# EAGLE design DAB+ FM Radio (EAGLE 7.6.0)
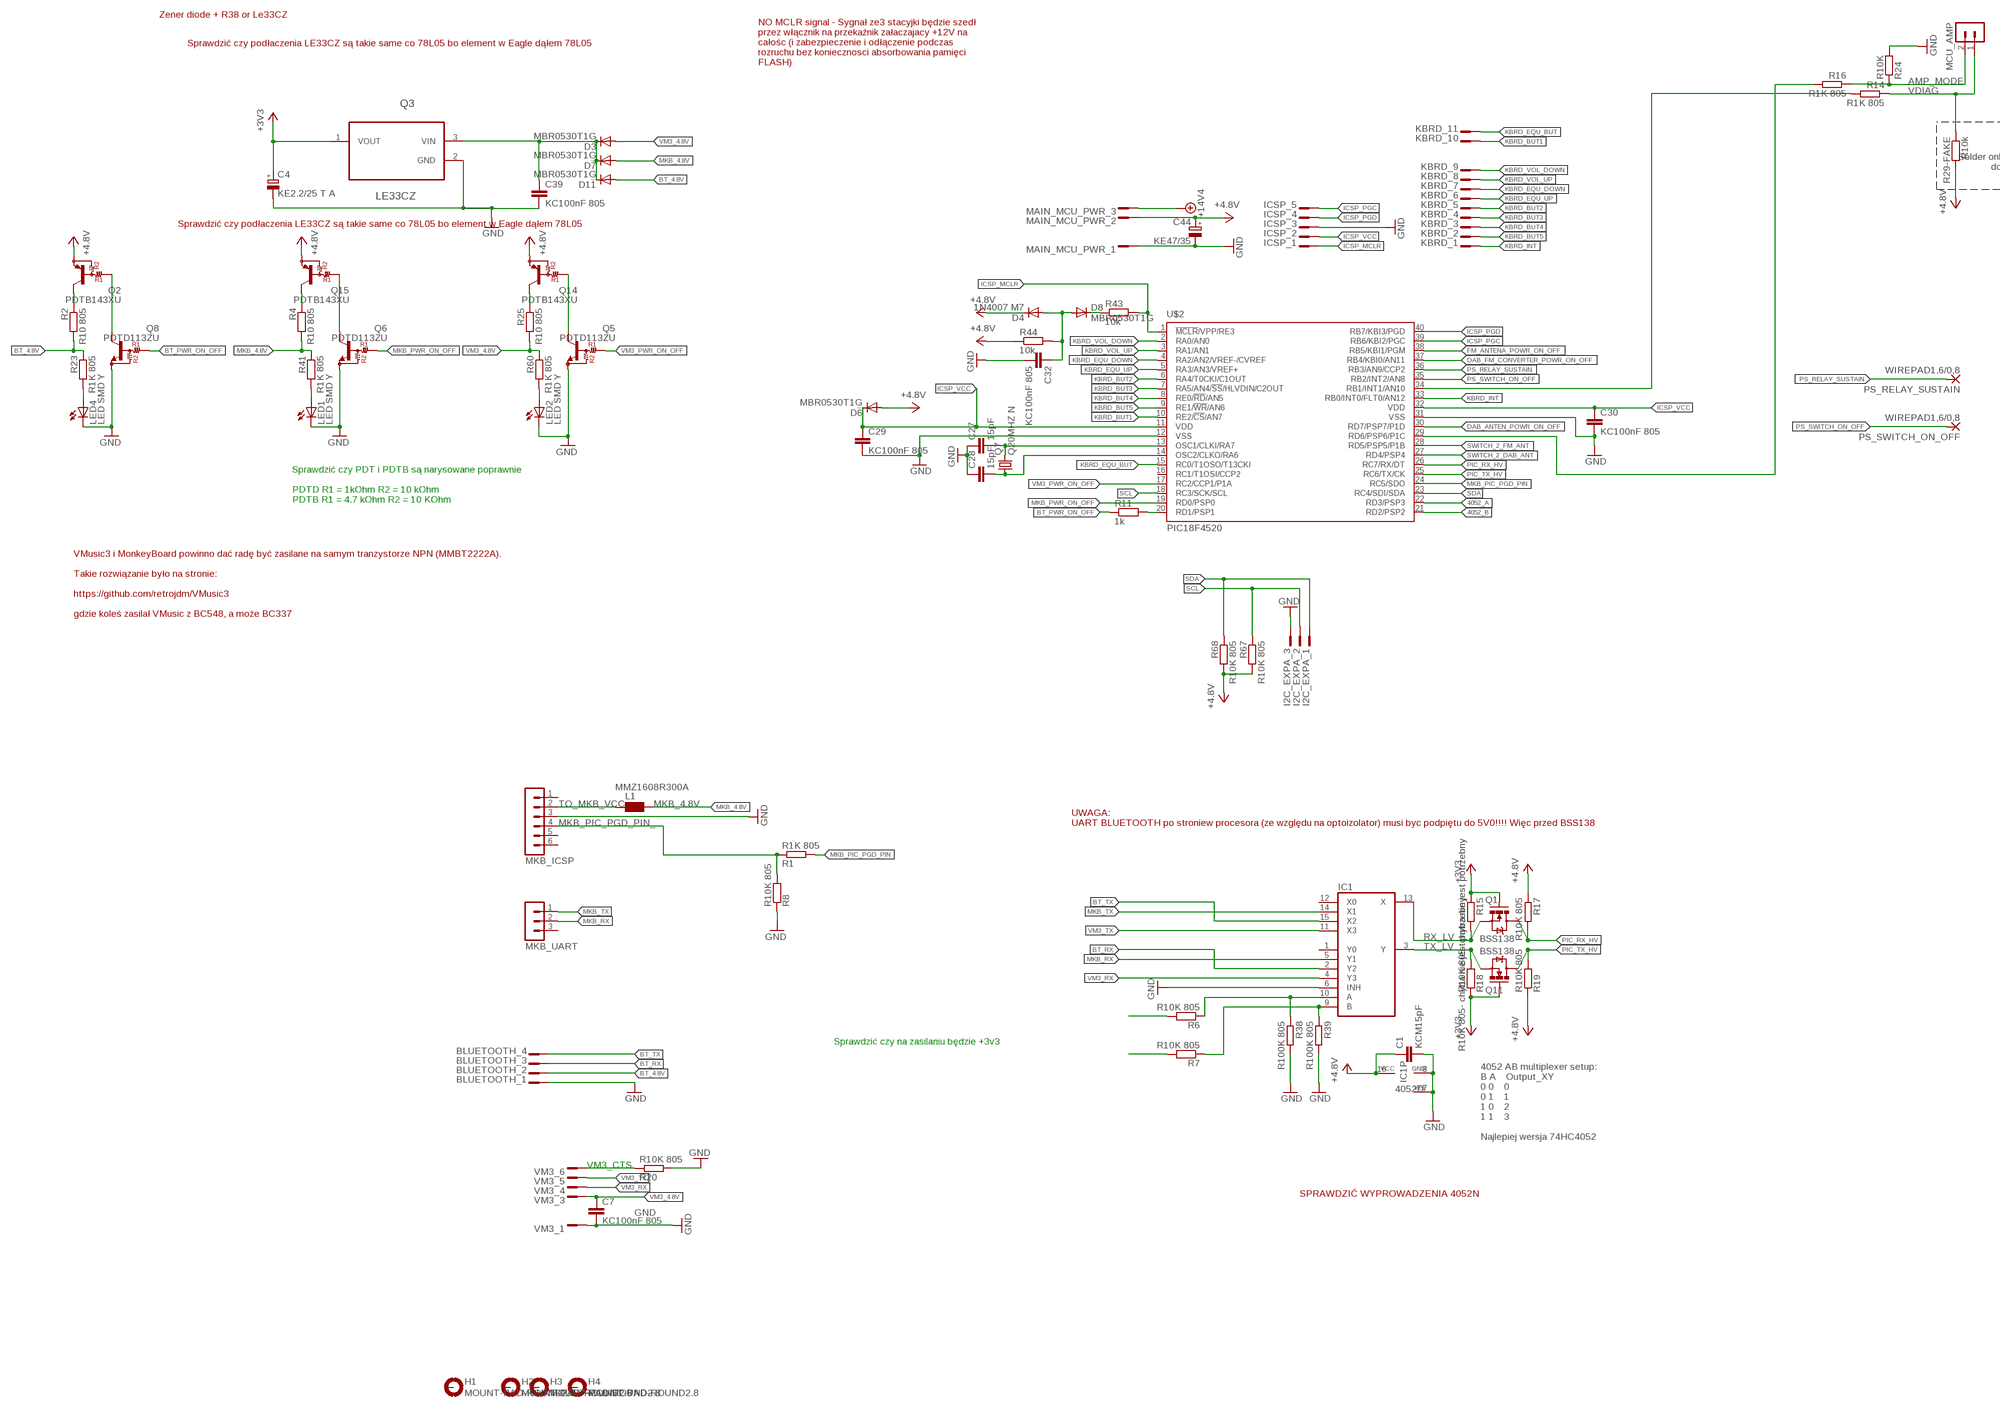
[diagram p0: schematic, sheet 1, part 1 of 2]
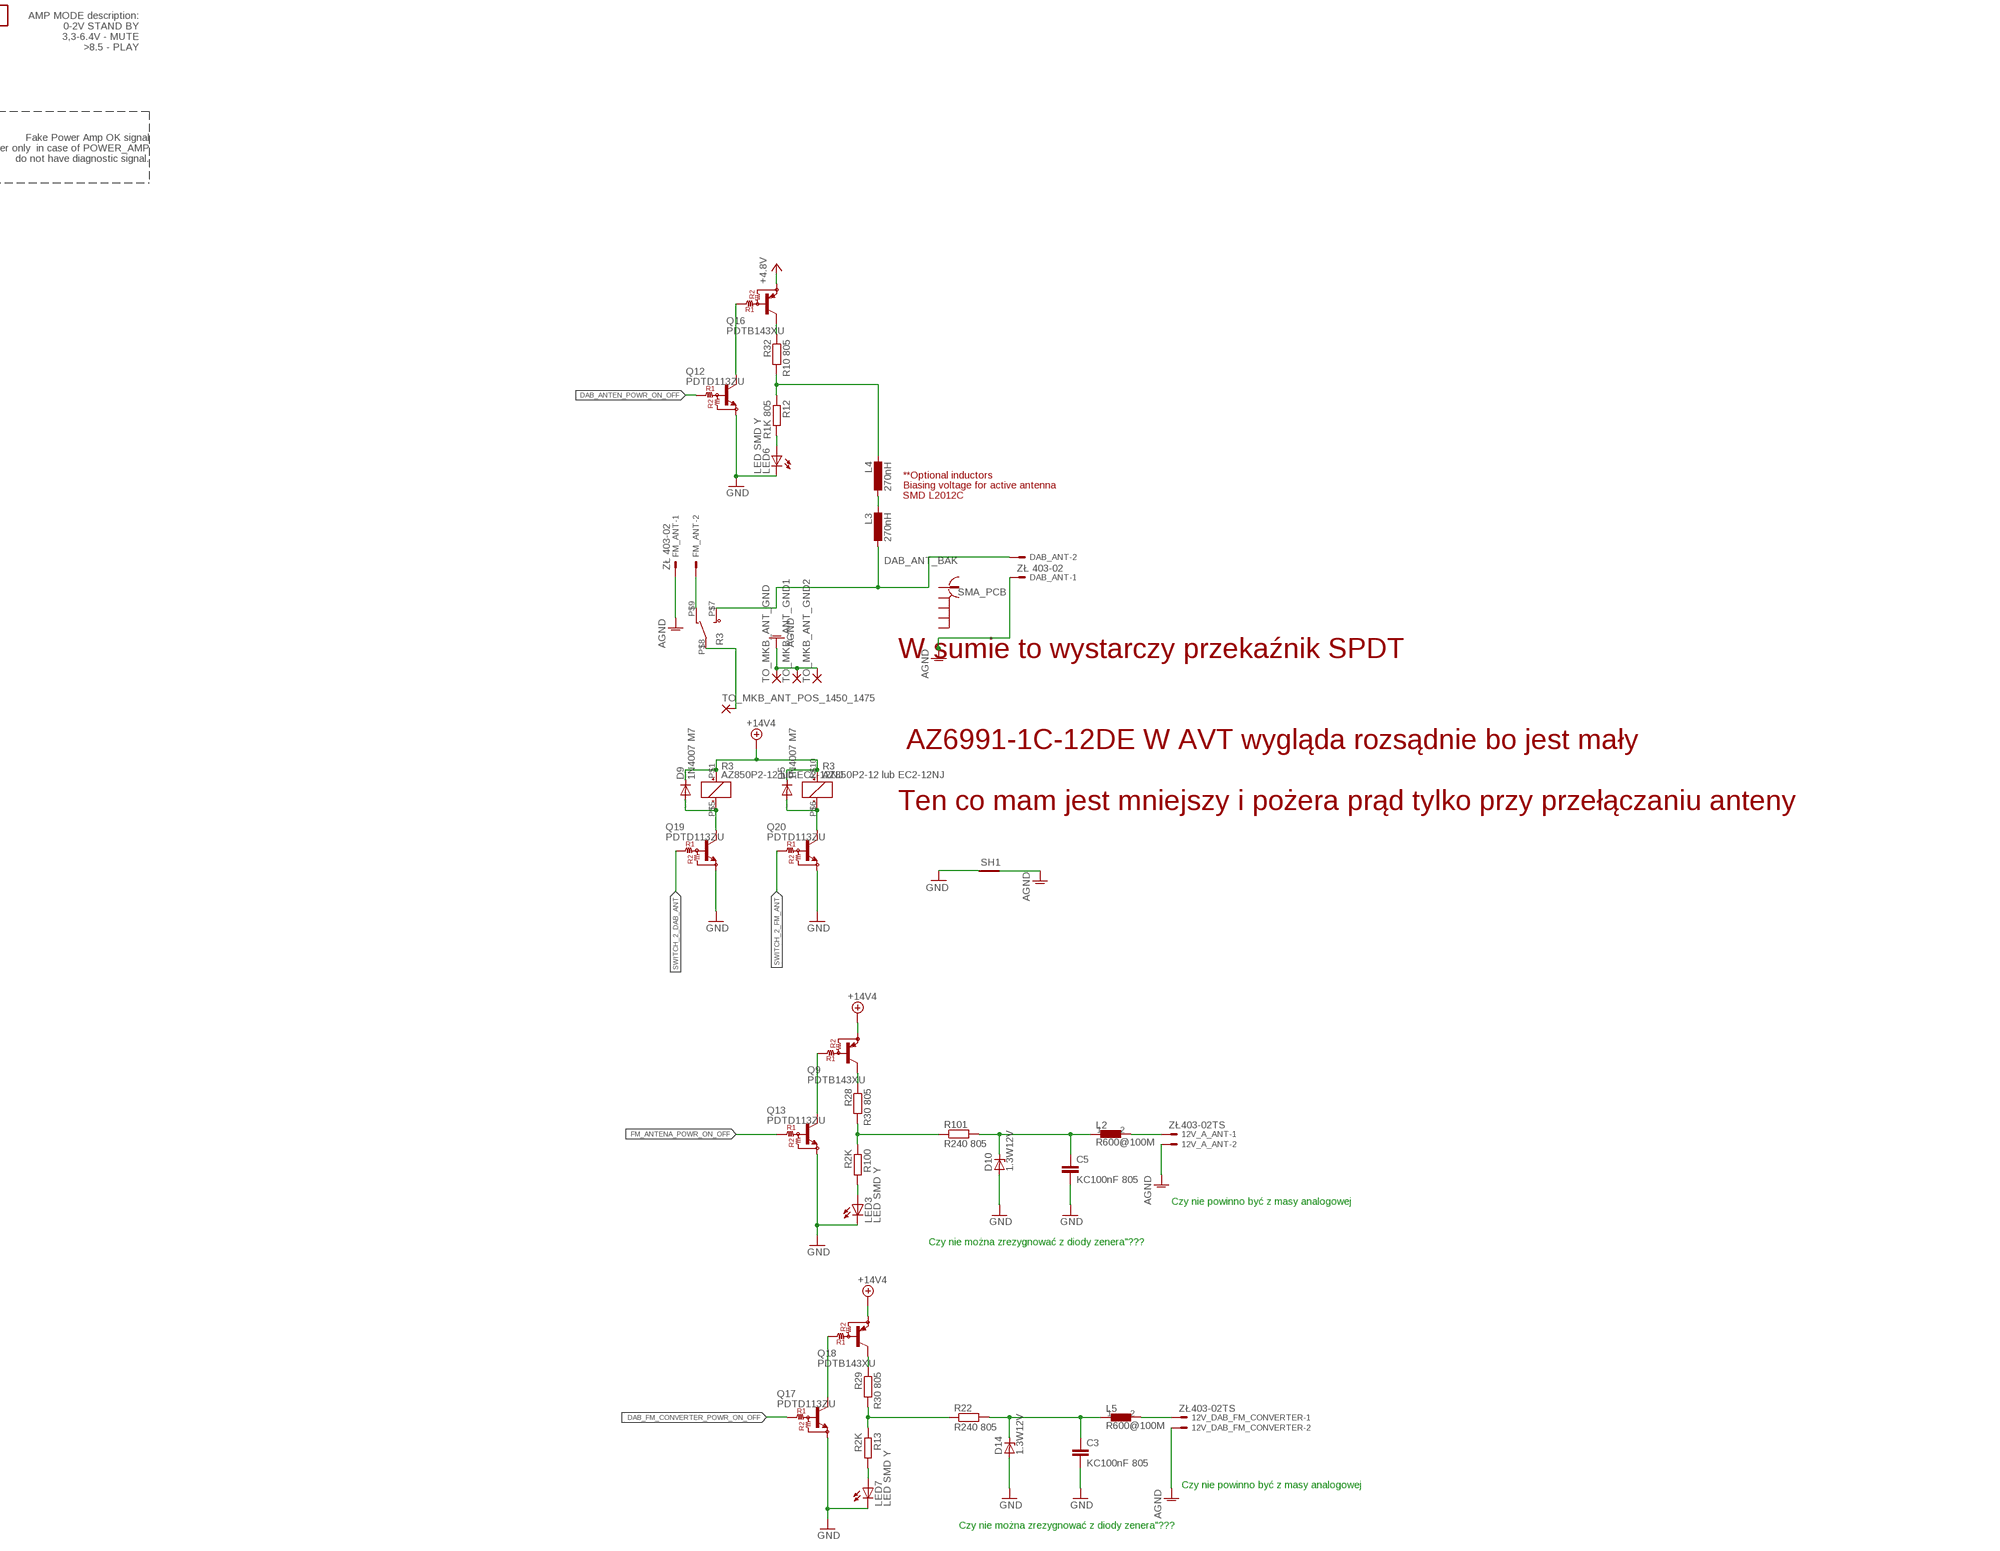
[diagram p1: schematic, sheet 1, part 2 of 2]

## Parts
12V_A_ANT  ZŁ403-02TS  22-23-2021  [22-23-2021]
12V_DAB_FM_CONVERTER  ZŁ403-02TS  22-23-2021  [22-23-2021]
BLUETOOTH  JST_4_PIN_B4B-PH-KS  [B4B-PH-KS]
C1  KCM15pF  C-EUC0805  [C0805]
C3  KC100nF 805  C-EUC0805  [C0805]
C4  KE2.2/25 T A  CPOL-EUSMCB  [SMC_B]
C5  KC100nF 805  C-EUC0805  [C0805]
C7  KC100nF 805  C-EUC0805  [C0805]
C27  15pF  C-EUC0805  [C0805]
C28  15pF  C-EUC0805  [C0805]
C29  KC100nF 805  C-EUC0805  [C0805]
C30  KC100nF 805  C-EUC0805  [C0805]
C32  KC100nF 805  C-EUC0805  [C0805]
C39  KC100nF 805  C-EUC0805  [C0805]
C44  KE47/35  CPOL-EUTT2D6  [TT2D6]
D3  MBR0530T1G  MBR0520LT  [SOD123]
D4  1N4007 M7  CGRM4001-G  [SOD-123_MINI-SMA]
D5  1N4007 M7  CGRM4001-G  [SOD-123_MINI-SMA]
D6  MBR0530T1G  MBR0520LT  [SOD123]
D7  MBR0530T1G  MBR0520LT  [SOD123]
D8  MBR0530T1G  MBR0520LT  [SOD123]
D9  1N4007 M7  CGRM4001-G  [SOD-123_MINI-SMA]
D10  1.3W12V  ZENER-DIODEZD-2.5  [ZDIO-2.5]
D11  MBR0530T1G  MBR0520LT  [SOD123]
D14  1.3W12V  ZENER-DIODEZD-2.5  [ZDIO-2.5]
DAB_ANT  ZŁ 403-02  22-27-2021-02  [6410-02]
DAB_ANT_BAK  SMA_PCB  [SMA_PCB]
FM_ANT  ZŁ 403-02  22-27-2021-02  [6410-02]
H1  MOUNT-PAD-ROUND2.8  [2,8-PAD]
H2  MOUNT-PAD-ROUND2.8  [2,8-PAD]
H3  MOUNT-PAD-ROUND2.8  [2,8-PAD]
H4  MOUNT-PAD-ROUND2.8  [2,8-PAD]
I2C_EXPA  JST_3_PIN_B3B-PH-KS  [B3B-PH-KS]
IC1  4052D  [SO16]
ICSP  JST_5_PIN_B5B-PH-KS  [B5B-PH-KS]
KBRD  JST_11_PIN_B11B-PH-KS  [B11B-PH-KS]
L1  MMZ1608R300A  WE-CBF_0603  [0603]
L2  R600@100M  FERRITR0805  [R0805]
L3  270nH  L-EUL2012C  [L2012C]
L4  270nH  L-EUL2012C  [L2012C]
L5  R600@100M  FERRITR0805  [R0805]
LED1  LED SMD Y  LEDCHIP-LED0805  [CHIP-LED0805]
LED2  LED SMD Y  LEDCHIP-LED0805  [CHIP-LED0805]
LED3  LED SMD Y  LED  [SMARTLED-TTW]
LED4  LED SMD Y  LEDCHIP-LED0805  [CHIP-LED0805]
LED6  LED SMD Y  LED  [SMARTLED-TTW]
LED7  LED SMD Y  LED  [SMARTLED-TTW]
MAIN_MCU_PWR  JST_3_PIN_B3B-XH-A  [B3B-XH-A]
MCU_AMP  MA02-1  [MA02-1]
MKB_ICSP  MA06-1  [MA06-1]
MKB_UART  MA03-1  [MA03-1]
PS_RELAY_SUSTAIN  WIREPAD1,6/0,8  [1,6/0,8]
PS_SWITCH_ON_OFF  WIREPAD1,6/0,8  [1,6/0,8]
Q1  BSS138  MOSFET-NCHANNELSMD  [SOT23-3]
Q2  PDTB143XU  [SOT-23]
Q3  LE33CZ  [TO127P254X749-3]
Q5  PDTD113ZU  [SOT-23]
Q6  PDTD113ZU  [SOT-23]
Q7  Q20MHZ N  CRYSTALHC49S  [HC49/S]
Q8  PDTD113ZU  [SOT-23]
Q9  PDTB143XU  [SOT-23]
Q11  BSS138  MOSFET-NCHANNELSMD  [SOT23-3]
Q12  PDTD113ZU  [SOT-23]
Q13  PDTD113ZU  [SOT-23]
Q14  PDTB143XU  [SOT-23]
Q15  PDTB143XU  [SOT-23]
Q16  PDTB143XU  [SOT-23]
Q17  PDTD113ZU  [SOT-23]
Q18  PDTB143XU  [SOT-23]
Q19  PDTD113ZU  [SOT-23]
Q20  PDTD113ZU  [SOT-23]
R1  R1K 805  R-EU_R0805  [R0805]
R2  R10 805  R-EU_R0805  [R0805]
R3  AZ850P2-12 lub EC2-12NJ  AZ850P2-12  [AZ850-2C]
R4  R10 805  R-EU_R0805  [R0805]
R6  R10K 805  R-EU_R0805  [R0805]
R7  R10K 805  R-EU_R0805  [R0805]
R8  R10K 805  R-EU_R0805  [R0805]
R11  1k  R-EU_R0805  [R0805]
R12  R1K 805  R-EU_R0805  [R0805]
R13  R2K  R-EU_R0805  [R0805]
R14  R1K 805  R-EU_R0805  [R0805]
R15  R10K 805- chyba nie jest potrzebny  R-EU_R0805  [R0805]
R16  R1K 805  R-EU_R0805  [R0805]
R17  R10K 805  R-EU_R0805  [R0805]
R18  R10K 805- chyba nie jest potrzebny  R-EU_R0805  [R0805]
R19  R10K 805  R-EU_R0805  [R0805]
R20  R10K 805  R-EU_R0805  [R0805]
R22  R240 805  R-EU_M0805  [M0805]
R23  R1K 805  R-EU_R0805  [R0805]
R24  R10K  R-EU_R0805  [R0805]
R25  R10 805  R-EU_R0805  [R0805]
R28  R30 805  R-EU_R0805  [R0805]
R29  R30 805  R-EU_R0805  [R0805]
R29-FAKE  R10k  R-EU_M0805  [M0805]
R32  R10 805  R-EU_R0805  [R0805]
R38  R100K 805  R-EU_M0805  [M0805]
R39  R100K 805  R-EU_M0805  [M0805]
R41  R1K 805  R-EU_R0805  [R0805]
R43  10k  R-EU_R0805  [R0805]
R44  10k  R-EU_M0805  [M0805]
R60  R1K 805  R-EU_R0805  [R0805]
R67  R10K 805  R-EU_R0805  [R0805]
R68  R10K 805  R-EU_R0805  [R0805]
R100  R2K  R-EU_R0805  [R0805]
R101  R240 805  R-EU_M0805  [M0805]
SH1  SHORT-HT5  [SHORT_TOP-50]
TO_MKB_ANT_GND  2,54/0,8  [2,54/0,8]
TO_MKB_ANT_GND1  2,54/0,8  [2,54/0,8]
TO_MKB_ANT_GND2  2,54/0,8  [2,54/0,8]
TO_MKB_ANT_POS_1450_1475  2,54/0,8  [2,54/0,8]
U$2  PIC18F4520  [DIL40]
VM3  JST_6_PIN_B6B-PH-KS  [B6B-PH-KS]

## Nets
4052_A: R6.2 U$2.22(RD3/PSP3)
4052_B: R7.2 U$2.21(RD2/PSP2)
+3V3: C4.+ Q1.1(G) Q3.1(VOUT) Q11.1(G) R15.1 R18.1
+5V: C1.1 C44.+ D4.C D6.A IC1.16(VCC) MAIN_MCU_PWR.P$2 Q2.2(E) Q14.2(E) Q15.2(E) Q16.2(E) R17.1 R19.1 R29-FAKE.2 R44.1 R67.2 R68.2 ; supply symbol labelled +4.8V
+14V4: D5.C D9.C MAIN_MCU_PWR.P$3 Q9.2(E) Q18.2(E) R3.P$1(S$1:+) R3.P$10(R$2:+)
AGND: 12V_A_ANT.2 12V_DAB_FM_CONVERTER.2 DAB_ANT.1 FM_ANT.1 SH1.2 TO_MKB_ANT_GND1.1(P) TO_MKB_ANT_GND2.1(P) TO_MKB_ANT_GND.1(P)
AMP_MODE: MCU_AMP.2 R16.1 R24.1
BT_4.8V: BLUETOOTH.P$2 D11.A R2.2 R23.1
BT_PWR_ON_OFF: Q8.1(B) R11.1
BT_RX: BLUETOOTH.P$3 IC1.2(Y2)
BT_TX: BLUETOOTH.P$4 IC1.15(X2)
DAB_ANTEN_POWR_ON_OFF: Q12.1(B) U$2.30(RD7/PSP7/P1D)
DAB_FM_CONVERTER_POWR_ON_OFF: Q17.1(B) U$2.37(RB4/KBI0/AN11)
FM_ANTENA_POWR_ON_OFF: Q13.1(B) U$2.38(RB5/KBI1/PGM)
GND: BLUETOOTH.P$1 C1.2 C3.2 C4.- C5.2 C7.2 C27.1 C28.1 C29.2 C30.2 C32.2 C39.2 C44.- D10.A D14.A I2C_EXPA.P$3 IC1.6(INH) IC1.7(VEE) IC1.8(GND) ICSP.P$3 LED1.C LED2.C LED3.C@1(C) LED4.C LED6.C@1(C) LED7.C@1(C) MAIN_MCU_PWR.P$1 MKB_ICSP.3 Q3.2(GND) Q5.2(E) Q6.2(E) Q8.2(E) Q12.2(E) Q13.2(E) Q17.2(E) Q19.2(E) Q20.2(E) R8.1 R20.2 R24.2 R38.2 R39.2 SH1.1 U$2.12(VSS) U$2.31(VSS) VM3.P$1
ICSP_MCLR: ICSP.P$1 R43.2 U$2.1(!MCLR!/VPP/RE3)
ICSP_PGC: ICSP.P$5 U$2.39(RB6/KBI2/PGC)
ICSP_PGD: ICSP.P$4 U$2.40(RB7/KBI3/PGD)
ICSP_VCC: C29.1 C30.1 D6.C ICSP.P$2 U$2.11(VDD) U$2.32(VDD)
KBRD_BUT1: KBRD.P$10 U$2.10(RE2/!CS!/AN7)
KBRD_BUT2: KBRD.P$5 U$2.6(RA4/T0CKI/C1OUT)
KBRD_BUT3: KBRD.P$4 U$2.7(RA5/AN4/!SS!/HLVDIN/C2OUT)
KBRD_BUT4: KBRD.P$3 U$2.8(RE0/!RD!/AN5)
KBRD_BUT5: KBRD.P$2 U$2.9(RE1/!WR!/AN6)
KBRD_EQU_BUT: KBRD.P$11 U$2.15(RC0/T1OSO/T13CKI)
KBRD_EQU_DOWN: KBRD.P$7 U$2.4(RA2/AN2/VREF-/CVREF)
KBRD_EQU_UP: KBRD.P$6 U$2.5(RA3/AN3/VREF+)
KBRD_INT: KBRD.P$1 U$2.33(RB0/INT0/FLT0/AN12)
KBRD_VOL_DOWN: KBRD.P$9 U$2.2(RA0/AN0)
KBRD_VOL_UP: KBRD.P$8 U$2.3(RA1/AN1)
MKB_4.8V: D7.A L1.2 R4.2 R41.1
MKB_PIC_PGD_PIN: R1.2 U$2.24(RC5/SDO)
MKB_PIC_PGD_PIN_: MKB_ICSP.4 R1.1 R8.2
MKB_PWR_ON_OFF: Q6.1(B) U$2.19(RD0/PSP0)
MKB_RX: IC1.5(Y1) MKB_UART.2
MKB_TX: IC1.14(X1) MKB_UART.1
N$1: L4.1 R12.1 R32.2
N$2: D9.A Q19.3(C) R3.P$5(S$1:-)
N$3: R3.P$8 TO_MKB_ANT_POS_1450_1475.1(P)
N$4: DAB_ANT.2 L3.2 R3.P$7
N$5: FM_ANT.2 R3.P$9
N$6: D5.A Q20.3(C) R3.P$6(R$2:-)
N$7: Q2.3(C) R2.1
N$8: R16.2 U$2.29(RD6/PSP6/P1C)
N$9: C39.1 D3.C D7.C D11.C Q3.3(VIN)
N$10: R14.2 U$2.34(RB1/INT1/AN10)
N$12: L3.1 L4.2
N$13: IC1.9(B) R7.1 R39.1
N$15: C27.2 Q7.2 U$2.13(OSC1/CLKI/RA7)
N$16: C28.2 Q7.1 U$2.14(OSC2/CLKO/RA6)
N$17: R11.2 U$2.20(RD1/PSP1)
N$18: Q15.3(C) R4.1
N$19: Q2.1(B) Q8.3(C)
N$20: Q12.3(C) Q16.1(B)
N$21: LED4.A R23.2
N$23: LED6.A@1(A) R12.2
N$25: Q17.3(C) Q18.1(B)
N$26: R13.1 R22.1 R29.2
N$27: LED7.A@1(A) R13.2
N$28: Q5.3(C) Q14.1(B)
N$29: C3.1 D14.C L5.1 R22.2
N$30: 12V_DAB_FM_CONVERTER.1 L5.2
N$31: LED2.A R60.2
N$32: Q14.3(C) R25.1
N$33: Q16.3(C) R32.1
N$34: Q9.3(C) R28.1
N$35: Q18.3(C) R29.1
N$37: Q6.3(C) Q15.1(B)
N$39: LED1.A R41.2
N$41: D8.C R43.1
N$42: C32.1 D4.A D8.A R44.2
N$44: R20.1 VM3.P$6
N$47: IC1.10(A) R6.1 R38.1
N$85: Q9.1(B) Q13.3(C)
N$87: R28.2 R100.1 R101.1
N$88: LED3.A@1(A) R100.2
N$91: C5.1 D10.C L2.1 R101.2
N$92: 12V_A_ANT.1 L2.2
PIC_RX_HV: Q1.3(D) R17.2 U$2.26(RC7/RX/DT)
PIC_TX_HV: Q11.3(D) R19.2 U$2.25(RC6/TX/CK)
PS_RELAY_SUSTAIN: PS_RELAY_SUSTAIN.1(P) U$2.36(RB3/AN9/CCP2)
PS_SWITCH_ON_OFF: PS_SWITCH_ON_OFF.1(P) U$2.35(RB2/INT2/AN8)
RX_LV: IC1.13(X) Q1.2(S) R15.2
SCL: I2C_EXPA.P$2 R67.1 U$2.18(RC3/SCK/SCL)
SDA: I2C_EXPA.P$1 R68.1 U$2.23(RC4/SDI/SDA)
SWITCH_2_DAB_ANT: Q19.1(B) U$2.27(RD4/PSP4)
SWITCH_2_FM_ANT: Q20.1(B) U$2.28(RD5/PSP5/P1B)
TO_MKB_VCC: L1.1 MKB_ICSP.2
TX_LV: IC1.3(Y) Q11.2(S) R18.2
VDIAG: MCU_AMP.1 R14.1 R29-FAKE.1
VM3_4.8V: C7.1 D3.A R25.2 R60.1 VM3.P$3
VM3_PWR_ON_OFF: Q5.1(B) U$2.17(RC2/CCP1/P1A)
VM3_RX: IC1.4(Y3) VM3.P$4
VM3_TX: IC1.11(X3) VM3.P$5
Unconnected: DAB_ANT_BAK.P$1 H1.B2,8(MOUNT) H2.B2,8(MOUNT) H3.B2,8(MOUNT) H4.B2,8(MOUNT) IC1.1(Y0) IC1.12(X0) MKB_ICSP.1 MKB_ICSP.5 MKB_ICSP.6 MKB_UART.3 R3.P$2 R3.P$3 R3.P$4 U$2.16(RC1/T1OSI/CCP2) VM3.P$2

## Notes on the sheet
- Zener diode + R38 or Le33CZ
- Sprawdzić czy podłaczenia LE33CZ są takie same co 78L05 bo element w Eagle dąłem 78L05
- NO MCLR signal - Sygnał ze3 stacyjki będzie szedł
  przez włącznik na przekaźnik załaczajacy +12V na
  całośc (i zabezpieczenie i odłączenie podczas
  rozruchu bez koniecznosci absorbowania pamięci
  FLASH)
- AMP MODE description:
  0-2V STAND BY
  3,3-6.4V - MUTE
  >8.5 - PLAY
- Fake Power Amp OK signal
  Solder only  in case of POWER_AMP
  do not have diagnostic signal.
- Sprawdzić czy podłaczenia LE33CZ są takie same co 78L05 bo element w Eagle dąłem 78L05
- **Optional inductors
- Biasing voltage for active antenna
- SMD L2012C
- Sprawdzić czy PDT i PDTB są narysowane poprawnie
  
  PDTD R1 = 1kOhm R2 = 10 kOhm
  PDTB R1 = 4.7 kOhm R2 = 10 KOhm
- VMusic3 i MonkeyBoard powinno dać radę być zasilane na samym tranzystorze NPN (MMBT2222A).
  
  Takie rozwiązanie było na stronie:
  
  https://github.com/retrojdm/VMusic3
  
  gdzie koleś zasilał VMusic z BC548, a może BC337
- W sumie to wystarczy przekaźnik SPDT
  
  
   AZ6991-1C-12DE W AVT wygląda rozsądnie bo jest mały
  
  Ten co mam jest mniejszy i pożera prąd tylko przy przełączaniu anteny
- UWAGA:
  UART BLUETOOTH po stroniew procesora (ze względu na optoizolator) musi byc podpiętu do 5V0!!!! Więc przed BSS138
- Sprawdzić czy na zasilaniu będzie +3v3
- 4052 AB multiplexer setup:
  B A    Output_XY
  0 0    0
  0 1    1
  1 0    2
  1 1    3
  
  Najlepiej wersja 74HC4052
- Czy nie powinno być z masy analogowej
- VM3_CTS
- Czy nie można zrezygnować z diody zenera"???
- SPRAWDZIĆ WYPROWADZENIA 4052N
- Czy nie powinno być z masy analogowej
- Czy nie można zrezygnować z diody zenera"???

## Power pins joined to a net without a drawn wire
GND: DAB_ANT_BAK.GND@1(GND) DAB_ANT_BAK.GND@2(GND) DAB_ANT_BAK.GND@3(GND) DAB_ANT_BAK.GND@4(GND)

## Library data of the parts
12V_A_ANT 12V_DAB_FM_CONVERTER = con-molex:22-23-2021: .100" (2.54mm) Center Header - 2 Pin; MF: MOLEX; MPN: 22-23-2021; OC_FARNELL: 1462926; OC_NEWARK: 25C3832
BLUETOOTH = conn-JST:JST_4_PIN_
C1 C3 C5 C7 C27-C30 C32 C39 = rcl:C-EU: CAPACITOR, European symbol
C4 = resistor:CPOL-EU: POLARIZED CAPACITOR, European symbol
C44 = rcl:CPOL-EU: POLARIZED CAPACITOR, European symbol
D3 D6-D8 D11 = diode:MBR0520LT: SCHOTTKY BARRIER RECTIFIER
D4 D5 D9 = diode:CGRM400*-G: Molded plasitc,JEDEC SOD-123/Mini SMA
D10 D14 = diode:ZENER-DIODE: Z-Diode
DAB_ANT FM_ANT = con-molex:22-?-02: CONNECTOR; OC_FARNELL: unknown; OC_NEWARK: unknown
DAB_ANT_BAK = Monkey:SMA_PCB: TE CONNECTIVITY - 5-1814832-1 - SOCKET, SMA, STRAIGHT PCB,50OHM Manufacturer: TE CONNECTIVITY Order Code: 1248990 Manufacturer Part No: 5-1814832-1 http://www.farnell.com/datasheets/316178.pdf
H1-H4 = holes:MOUNT-PAD-ROUND: MOUNTING PAD, round
I2C_EXPA MAIN_MCU_PWR = conn-JST:JST_3_PIN_
IC1 = 40xx:4052: Dual 4-channel ANALOG MULTIPLEXER
ICSP = conn-JST:JST_5_PIN_
KBRD = conn-JST:JST_11_PIN_
L1 = wuerth-elektronik:WE-CBF: SMD EMI Suppression Ferrite Beads
L2 L5 = ferrit_bear:FERRIT
L3 L4 = resistor:L-EU: INDUCTOR, European symbol
LED1-LED4 LED6 LED7 = adafruit:LED: LED
MCU_AMP = con-lstb_SileliS:MA02-1: PIN HEADER
MKB_ICSP = con-lstb:MA06-1: PIN HEADER; OC_FARNELL: unknown; OC_NEWARK: unknown
MKB_UART = con-lstb:MA03-1: PIN HEADER; OC_FARNELL: unknown; OC_NEWARK: unknown
PS_RELAY_SUSTAIN PS_SWITCH_ON_OFF = wirepad:WIREPAD: Wire PAD connect wire on PCB
Q1 Q11 = SparkFun:MOSFET-NCHANNEL
Q2 Q9 Q14-Q16 Q18 = pre-bias-transistor:PDTB: PNP Resistor-Equipped Transistor (RET) family in a very small SOT323 (SC-70) Surface-Mounted Device (SMD) plastic package. VCC = -50 IC (max) = -500mA; R1: 4.7 kOhm; R2: 10 kOhm
Q3 = LE33cz:LE33CZ: VOLTAGE REGULATORS; MPN: LE33CZ; OC_FARNELL: 9755349; OC_NEWARK: 26M0166; PACKAGE: TO-92; SUPPLIER: STMICROELECTRONICS
Q5 Q6 Q8 Q12 Q13 Q17 Q19 Q20 = pre-bias-transistor:PDTD: Pre biase NPN transistor NPN Resistor-Equipped Transistor (RET) family in a very small SOT323 (SC-70) Surface-Mounted Device (SMD) plastic package. VCC = 50V Ic (max) = 500 mA; R1: 1 kOhm; R2: 10 kOhm
Q7 = adafruit:CRYSTAL: CRYSTAL; OC_FARNELL: 1667008; OC_NEWARK: unknown
R1 R2 R4 R6-R8 R11-R20 R22-R25 R28 R29 R29-FAKE R32 R38 R39 R41 R43 R44 R60 R67 R68 R100 R101 = rcl:R-EU_: RESISTOR, European symbol
R3 = relay_silelis:AZ850P2-12
SH1 = shorts-old:SHORT-H: Short between two nets; BOM: no
TO_MKB_ANT_GND TO_MKB_ANT_GND1 TO_MKB_ANT_GND2 TO_MKB_ANT_POS_1450_1475 = wirepad:2,54/0,8: THROUGH-HOLE PAD
U$2 = microchip_SileliS:PIC18F4*20
VM3 = conn-JST:JST_6_PIN_

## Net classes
1 VCC: width 0.6 mm, clearance 0.6 mm

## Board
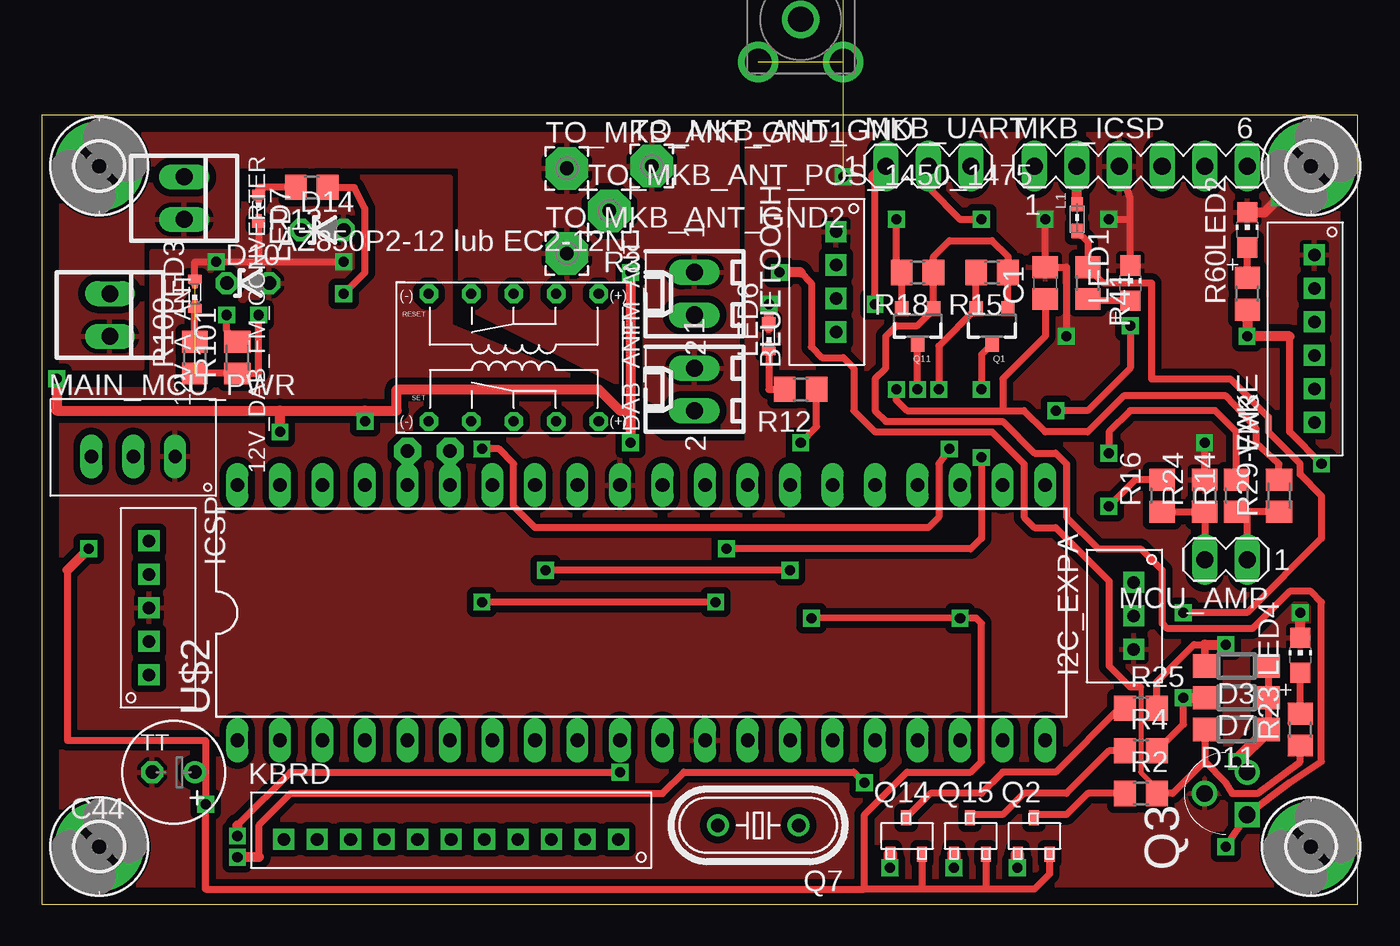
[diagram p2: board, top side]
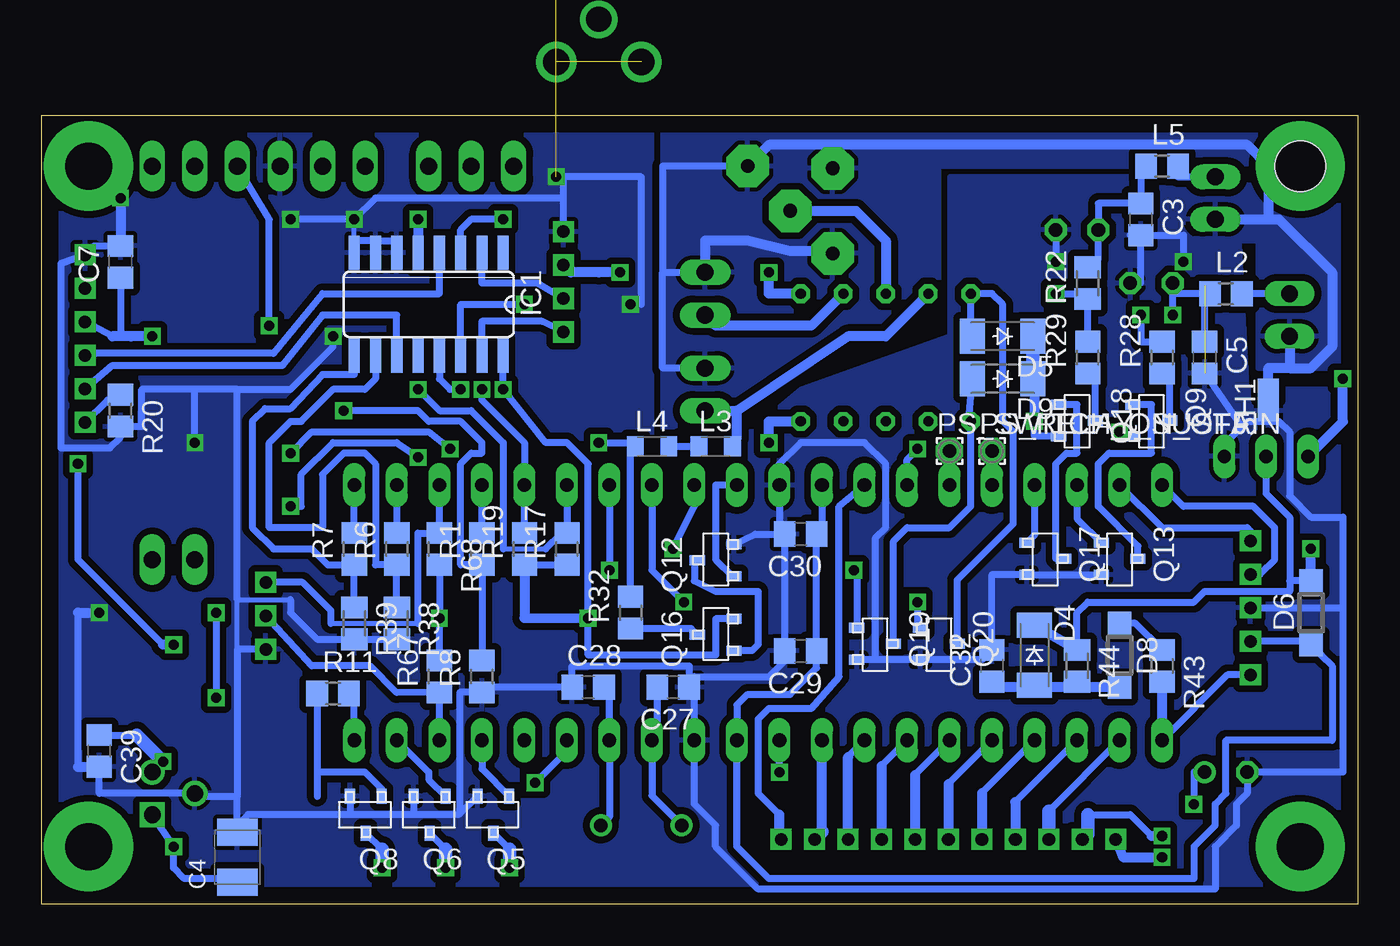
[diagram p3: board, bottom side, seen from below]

Size 78.61 x 47.12 mm. Coordinates in mm from the lower left corner, seen from the top.
Outline: 0,0 78.61,0 78.61,47.12 0,47.12 0,0
Copper layers (1*16): Top 0.035mm / dielectric 1.5mm / Bottom 0.035mm
Design rules "default": minimum track width 10mil, minimum drill 24mil, track to track 8mil, track to pad 8mil, pad to pad 8mil, via to via 8mil, smd to smd 8mil, copper to edge 40mil, drill to drill 8mil, minimum pad ring 10mil, minimum via ring 8mil, stop-mask expansion 4mil, vias tented up to drill 0mil, thermal gap 10mil
Holes 3 mm at 3.43,44.07

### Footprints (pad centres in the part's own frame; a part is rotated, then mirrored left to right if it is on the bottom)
22-23-2021 = drill 1 long: 1 -1.27,0; 2 1.27,0
B4B-PH-KS = drill 0.75 pad 1.2 square: P$1 -2,1.7; P$2 -4,1.7; P$3 -6,1.7; P$4 -8,1.7
C0805 = smd 1.3 x 1.5: 1 -0.95,0; 2 0.95,0
SMC_B = smd 1.6 x 2.4: + -1.5,0; - 1.5,0
TT2D6 = drill 0.813: + -1.27,0 | drill 0.813 octagon: - 1.27,0
SOD123 = smd 1.4 x 1.4: A 1.9,0; C -1.9,0
SOD-123_MINI-SMA = smd 1.5 x 2.1: A 1.8,0; C -1.8,0
ZDIO-2.5 = drill 0.813 octagon: A 1.27,0; C -1.27,0
6410-02 = drill 1.016 long: 1 1.27,0; 2 -1.27,0
SMA_PCB = drill 1.6: GND@1 -2.54,2.54; GND@2 2.54,2.54; GND@3 -2.54,-2.54; GND@4 2.54,-2.54 | drill 1.5: P$1 0,0
2,8-PAD = drill 2.8 pad 5.334: B2,8 0,0
B3B-PH-KS = drill 0.75 pad 1.2 square: P$1 -2,1.7; P$2 -4,1.7; P$3 -6,1.7
SO16 = smd 0.66 x 2.032: 1 -4.445,-3.073; 2 -3.175,-3.073; 3 -1.905,-3.073; 4 -0.635,-3.073; 5 0.635,-3.073; 6 1.905,-3.073; 7 3.175,-3.073; 8 4.445,-3.073; 9 4.445,3.073; 10 3.175,3.073; 11 1.905,3.073; 12 0.635,3.073; 13 -0.635,3.073; 14 -1.905,3.073; 15 -3.175,3.073; 16 -4.445,3.073
B5B-PH-KS = drill 0.75 pad 1.2 square: P$1 -2,1.7; P$2 -4,1.7; P$3 -6,1.7; P$4 -8,1.7; P$5 -10,1.7
B11B-PH-KS = drill 0.75 pad 1.2 square: P$1 -2,1.7; P$2 -4,1.7; P$3 -6,1.7; P$4 -8,1.7; P$5 -10,1.7; P$6 -12,1.7; P$7 -14,1.7; P$8 -16,1.7; P$9 -18,1.7; P$10 -20,1.7; P$11 -22,1.7
0603 = smd 0.85 x 0.7: 1 -0.9,0; 2 0.7,0
R0805 = smd 1.3 x 1.5: 1 -0.95,0; 2 0.95,0
L2012C = smd 1 x 1.2: 1 -1,0; 2 1,0
CHIP-LED0805 = smd 1.2 x 1.2: A 0,-1.05; C 0,1.05
SMARTLED-TTW = smd 0.8 x 0.5: A 0,-0.875; C 0,0.875 | smd 0.35 x 0.35: A@1 0,-0.5; C@1 0,0.5
B3B-XH-A = drill 0.8 long: P$1 -2.45,2.35; P$2 -4.95,2.35; P$3 -7.45,2.35
MA02-1 = drill 1.016 long: 1 -2.54,0; 2 0,0
MA06-1 = drill 1.016 long: 1 -6.35,0; 2 -3.81,0; 3 -1.27,0; 4 1.27,0; 5 3.81,0; 6 6.35,0
MA03-1 = drill 1.016 long: 1 -2.54,0; 2 0,0; 3 2.54,0
1,6/0,8 = drill 0.813 pad 1.6 octagon: 1 0,0
SOT23-3 = smd 0.8 x 0.9: 1 -0.95,-1; 2 0.95,-1; 3 0,1.1
SOT-23 = smd 0.6 x 0.9: 1 -1,-1.1; 2 0.9,-1.1; 3 -0.05,1.1
TO127P254X749-3 = drill 0.991 square: 1 -2.54,-2.54 | drill 0.991: 2 -1.27,0; 3 0,-2.54
HC49/S = drill 0.813: 1 -2.413,0; 2 2.413,0
AZ850-2C = drill 0.6 octagon: P$1 -5.08,3.81; P$2 -2.54,3.81; P$3 0,3.81; P$4 2.54,3.81; P$5 5.08,3.81; P$6 5.08,-3.81; P$7 2.54,-3.81; P$8 0,-3.81; P$9 -2.54,-3.81; P$10 -5.08,-3.81
M0805 = smd 1.3 x 1.6: 1 -0.95,0; 2 0.95,0
SHORT_TOP-50 = smd 1.27 x 1.27: 1 0.635,0; 2 -0.635,0
2,54/0,8 = drill 0.813 pad 2.54 octagon: 1 0,0
DIL40 = drill 0.813 long: 1 -24.13,-7.62; 2 -21.59,-7.62; 3 -19.05,-7.62; 4 -16.51,-7.62; 5 -13.97,-7.62; 6 -11.43,-7.62; 7 -8.89,-7.62; 8 -6.35,-7.62; 9 -3.81,-7.62; 10 -1.27,-7.62; 11 1.27,-7.62; 12 3.81,-7.62; 13 6.35,-7.62; 14 8.89,-7.62; 15 11.43,-7.62; 16 13.97,-7.62; 17 16.51,-7.62; 18 19.05,-7.62; 19 21.59,-7.62; 20 24.13,-7.62; 21 24.13,7.62; 22 21.59,7.62; 23 19.05,7.62; 24 16.51,7.62; 25 13.97,7.62; 26 11.43,7.62; 27 8.89,7.62; 28 6.35,7.62; 29 3.81,7.62; 30 1.27,7.62; 31 -1.27,7.62; 32 -3.81,7.62; 33 -6.35,7.62; 34 -8.89,7.62; 35 -11.43,7.62; 36 -13.97,7.62; 37 -16.51,7.62; 38 -19.05,7.62; 39 -21.59,7.62; 40 -24.13,7.62
B6B-PH-KS = drill 0.75 pad 1.2 square: P$1 -2,1.7; P$2 -4,1.7; P$3 -6,1.7; P$4 -8,1.7; P$5 -10,1.7; P$6 -12,1.7

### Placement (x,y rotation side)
12V_A_ANT  4.06,35.18 270 top
12V_DAB_FM_CONVERTER  8.51,42.16 270 top
BLUETOOTH  49.15,42.16 90 top
C1  59.94,37.08 90 top
C3  12.95,40.89 270 bottom
C4  66.93,2.79 90 bottom
C5  9.14,32.64 270 bottom
C7  73.91,38.35 90 bottom
C27  40.89,12.95 180 bottom
C28  45.97,12.95 0 bottom
C29  33.27,15.11 180 bottom
C30  33.27,22.1 180 bottom
C32  21.84,14.22 90 bottom
C39  75.18,9.14 270 bottom
C44  7.87,7.87 180 top
D3  71.37,14.22 180 top
D4  19.3,14.86 270 bottom
D5  21.21,33.91 180 bottom
D6  2.79,17.4 90 bottom
D7  71.37,12.32 180 top
D8  14.22,14.86 270 bottom
D9  21.21,31.37 180 bottom
D10  12.32,37.08 0 top
D11  71.37,10.41 180 top
D14  16.76,40.26 0 top
DAB_ANT  38.99,30.73 90 top
DAB_ANT_BAK  not placed on the board
FM_ANT  38.99,36.45 90 top
H1  75.82,44.07 0 top
H2  3.43,44.07 0 top
H3  3.43,3.43 0 top
H4  75.82,3.43 0 top
I2C_EXPA  66.93,21.21 90 top
IC1  55.5,35.81 180 bottom
ICSP  4.7,11.68 270 top
KBRD  36.45,2.16 0 top
L1  61.85,40.89 270 top
L2  7.87,36.45 0 bottom
L3  38.35,27.33 0 bottom
L4  42.16,27.33 0 bottom
L5  11.68,44.07 0 bottom
LED1  65.02,37.08 0 top
LED2  72.01,40.26 0 top
LED3  9.14,36.45 0 top
LED4  75.18,14.86 0 top
LED6  43.43,33.91 0 top
LED7  12.95,41.53 180 top
MAIN_MCU_PWR  10.41,24.38 0 top
MCU_AMP  69.47,20.57 180 top
MKB_ICSP  65.66,44.07 0 top
MKB_UART  52.96,44.07 0 top
PS_RELAY_SUSTAIN  21.84,27.05 0 bottom
PS_SWITCH_ON_OFF  24.38,27.05 0 bottom
Q1  56.77,34.54 180 top
Q2  59.31,4.06 0 top
Q3  69.47,7.87 90 top
Q5  51.69,5.33 180 bottom
Q6  55.5,5.33 180 bottom
Q7  42.8,4.7 180 top
Q8  59.31,5.33 180 bottom
Q9  12.32,28.83 270 bottom
Q11  52.32,34.54 180 top
Q12  38.35,20.57 90 bottom
Q13  14.22,20.57 270 bottom
Q14  51.69,4.06 0 top
Q15  55.5,4.06 0 top
Q16  38.35,16.13 90 bottom
Q17  18.67,20.57 270 bottom
Q18  16.76,28.83 270 bottom
Q19  28.83,15.49 270 bottom
Q20  25.02,15.49 270 bottom
R1  52.32,21.21 90 bottom
R2  65.66,6.6 0 top
R3  28.19,32.64 180 top
R4  65.66,9.14 0 top
R6  57.4,21.21 90 bottom
R7  59.94,21.21 90 bottom
R8  52.32,13.59 90 bottom
R11  61.21,12.57 0 bottom
R12  45.34,30.73 180 top
R13  16.13,42.8 180 top
R14  71.37,24.38 90 top
R15  56.77,37.72 180 top
R16  66.93,24.38 90 top
R17  47.24,21.21 90 bottom
R18  52.32,37.72 180 top
R19  49.78,21.21 90 bottom
R20  73.91,29.46 270 bottom
R22  16.13,37.08 90 bottom
R23  75.18,10.41 90 top
R24  69.47,24.38 90 top
R25  65.66,11.68 0 top
R28  11.68,32.64 90 bottom
R29  16.13,32.64 90 bottom
R29-FAKE  73.91,24.38 90 top
R32  43.43,17.4 90 bottom
R38  57.4,16.76 270 bottom
R39  59.94,16.76 270 bottom
R41  62.48,37.08 270 top
R43  11.68,14.22 270 bottom
R44  16.76,14.22 270 bottom
R60  72.01,36.45 90 top
R67  54.86,13.59 90 bottom
R68  54.86,21.21 270 bottom
R100  9.14,32.64 90 top
R101  11.68,32.64 90 top
SH1  5.33,30.1 270 bottom
TO_MKB_ANT_GND  36.45,44.07 0 top
TO_MKB_ANT_GND1  31.37,43.94 0 top
TO_MKB_ANT_GND2  31.37,38.86 0 top
TO_MKB_ANT_POS_1450_1475  33.91,41.4 0 top
U$2  35.81,17.4 0 top
VM3  77.72,40.77 90 top

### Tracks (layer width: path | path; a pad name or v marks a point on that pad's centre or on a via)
4052_A
  Bottom 0.406: U$2.22 R6.2
4052_B
  Bottom 0.406: R7.2 U$2.21
+3V3  (via drill 0.6)
  Top 0.406: Q1.1 R15.1 57.72,38.67 56.77,39.62 54.23,39.62 53.27,38.67 R18.1 Q11.1 53.27,35.49 52.32,34.54 51.05,34.54 50.42,33.91 50.42,32 49.78,31.37 49.78,29.46 50.42,28.83 57.4,28.83 59.31,26.92 60.58,26.92 61.21,26.29 61.21,23.11 63.12,21.21 65.66,21.21 66.93,19.94 66.93,16.76 67.25,16.45 72.33,16.45 74.55,18.67 75.82,18.67 76.45,18.03 76.45,8.51 74.55,7.24 Q3.1 v70.74,3.43
  Bottom 0.406: C4.+ 67.16,1.52 70.1,1.52 70.74,2.16 v70.74,3.43 Q3.1
+5V  (via drill 0.6)
  Top 0.406: v51.05,30.73 51.05,30.1 51.69,29.46 57.4,29.46 | 57.4,29.46 58.67,29.46 59.94,28.19 62.48,28.19 64.64,30.35 70.74,30.35 72.52,28.45 72.52,27.56 73.91,26.29 R29-FAKE.2 | Q14.2 52.59,0.89 | Q2.2 60.21,1.79 59.31,0.89 56.4,0.89 | 56.4,0.89 52.59,0.89 | 52.59,0.89 49.15,0.89 | Q15.2 56.4,0.89 | 49.15,0.89 49.15,5.33 51.69,7.87 55.5,7.87 56.13,8.51 56.13,16.76 55.83,17.07 v54.86,17.07 54.86,17.08 v45.97,17.07 | 1.52,19.94 1.52,9.78 9.78,9.78 v9.78,5.97 9.78,0.89 49.15,0.89 | C1.1 59.94,33.91 57.4,31.37 57.4,29.46
  Top 0.61: v2.79,21.21 1.52,19.94
  Bottom 0.406: IC1.16 v51.05,30.73 48.51,27.56 47.24,27.56 45.97,26.29 v45.97,17.07 45.97,14.86 38.35,14.86 38.35,17.03 Q16.2 | R19.1 R17.1 | R68.2 v54.86,17.07 R67.2 | 4.06,19.3 4.06,23.11 5.46,24.51 MAIN_MCU_PWR.P$2 | D6.A 4.06,19.3 | R44.1 16.76,17.4 16.13,18.03 9.78,18.03 9.14,18.67 4.06,18.67 4.06,19.3 | C44.+ 9.78,7.87 v9.78,5.97
  Bottom 0.61: R44.1 D4.C | D6.A v2.79,21.21 | R19.1 49.78,17.08 v45.97,17.07
+14V4  (via drill 0.6)
  Top 0.61: v0.89,31.37 0.89,29.46 14.22,29.46 | 14.22,29.46 19.3,29.46 | v19.3,28.83 19.3,29.46 | v35.18,37.72 35.18,29.46 | 35.18,29.46 v35.18,27.56 | 19.3,29.46 21.21,29.46 21.21,30.73 33.27,30.73 34.54,29.46 35.18,29.46 | v14.22,28.19 14.22,29.46
  Bottom 0.406: Q18.2 19.3,27.93 v19.3,28.83 | Q9.2 14.22,27.93 v14.22,28.19
  Bottom 0.61: MAIN_MCU_PWR.P$3 0.89,28.81 v0.89,31.37 | v35.18,27.56 35.18,28.83 R3.P$1 | R3.P$10 35.18,36.45 v35.18,37.72 | D9.C arc90 19.3,31.26 v19.3,28.83
  Bottom 0.813: D9.C D5.C
AGND
  Bottom 0.406: TO_MKB_ANT_GND.1 41.53,44.07 41.53,37.72 | 41.53,37.72 FM_ANT.1 | DAB_ANT.1 41.53,32 41.53,37.72
  Bottom 0.61: 31.37,45.34 6.6,45.34 5.33,44.07 5.33,40.89 | 31.37,45.34 35.18,45.34 TO_MKB_ANT_GND.1 | SH1.2 5.33,32 4.06,32 | TO_MKB_ANT_GND1.1 31.37,45.34 | TO_MKB_ANT_GND2.1 31.5,38.99 33.91,38.99 36.45,39.62 38.99,39.62 FM_ANT.1 | 5.33,40.89 4.7,40.89 1.52,37.72 1.52,33.27 2.79,32 4.06,32 | 12V_DAB_FM_CONVERTER.2 5.33,40.89 | 12V_A_ANT.2 4.06,32
  pour Bottom (isolate 0.406): -1.02,32 -0.38,46.61 41.53,46.61 41.53,28.19 25.02,35.81 25.02,44.07 11.68,44.07 11.68,39.62 5.97,39.62 5.97,32
  pour Top (isolate 0.406): -1.02,32 -1.02,46.61 41.53,46.61 41.53,28.19 37.72,29.46 25.02,35.81 25.02,44.07 11.68,44.07 11.68,39.62 5.97,39.62 5.97,32
AMP_MODE
  Top 0.406: R16.1 R24.1 MCU_AMP.2
BT_4.8V  (via drill 0.6)
  Top 0.305: 65.66,12.95 65.66,7.87 66.93,6.6
  Top 0.406: 67.09,7.08 R2.2 66.93,6.6 67.56,6.6 69.47,8.51 | D11.A 69.47,8.51 | R23.1 75.18,8.51 72.64,6.6 71.12,6.6 70.74,7.24 69.47,8.51 | 65.66,12.95 65.02,12.95 63.75,14.22 63.75,19.3 60.58,22.48 59.31,22.48 58.67,23.11 58.67,26.29 56.77,28.19 49.78,28.19 48.51,29.46 48.51,32 47.88,32.64 46.61,32.64 45.97,33.27 45.97,37.08 45.34,37.72
  Top 0.61: 45.34,37.72 v44.07,37.72
  Bottom 0.406: 47,37.72 BLUETOOTH.P$2 | 45.65,37.72 45.34,37.72
  Bottom 0.61: v44.07,37.72 45.34,37.72 47,37.72
BT_PWR_ON_OFF
  Bottom 0.406: R11.1 62.16,7.87 | 62.16,7.87 62.16,6.43 | 62.16,7.87 59.31,7.87 58.31,6.87 Q8.1
BT_RX
  Bottom 0.406: BLUETOOTH.P$3 49,37.08 52.32,37.08 IC1.2
BT_TX
  Bottom 0.406: IC1.15 52.32,34.8 48.72,34.8 BLUETOOTH.P$4
DAB_ANTEN_POWR_ON_OFF
  Bottom 0.406: U$2.30 38.35,25.02 38.35,20.57 37.35,19.57 Q12.1
DAB_FM_CONVERTER_POWR_ON_OFF
  Bottom 0.406: U$2.37 19.3,22.04 Q17.1
FM_ANTENA_POWR_ON_OFF
  Bottom 0.406: U$2.38 16.76,23.01 Q13.1
GND  (via drill 0.6)  (5 unrouted)
  Top 0.406: v59.94,40.89 C1.2 61.21,38.03 v61.21,33.91 | LED1.C 65.02,40.89 | MKB_ICSP.3 65.02,42.16 65.02,40.89 | v63.75,40.89 65.02,40.89 | R24.2 v69.47,27.56 | LED3.C@1 9.14,38.35 v10.41,38.35 12.95,38.35 | 12.95,38.35 v18.03,38.35 | LED7.C@1 12.95,38.35
  Top 0.61: LED4.C v75.18,17.4 | LED2.C 73.06,41.31 v73.91,42.16 | LED6.C@1 v43.43,35.81
  Bottom 0.305: IC1.8 59.94,39.62 v59.94,40.89 | 66.93,15.21 66.93,18.19 63.75,18.19
  Bottom 0.406: R38.2 R39.2 62.17,15.81 63.75,17.4 63.75,18.19 | 47.45,42.16 58.67,42.16 v59.94,40.89 v63.75,40.89 | IC1.6 57.4,39.62 58.67,39.62 | 58.67,39.62 59.94,39.62 | IC1.7 58.67,39.62 | 66.93,18.19 66.93,30.73 | 66.93,30.73 69.47,30.73 | 69.47,30.73 72.64,30.73 72.64,28.51 R20.2 73.91,27.88 74.55,27.24 77.47,27.24 77.47,38.26 VM3.P$1 75.49,39.3 C7.2 73.91,39.53 | Q5.2 53.64,5.38 | 53.64,5.38 53.69,5.33 56.4,5.33 | 56.4,5.33 60.21,5.33 | Q8.2 60.21,5.33 | Q6.2 56.4,5.33 | 66.93,6.43 69.93,6.43 Q3.2 75.18,6.6 C39.2 | C4.- 66.93,4.7 | 66.93,4.7 66.93,6.43 | 76.45,8.19 76.45,17.4 | 66.93,30.73 63.75,30.73 61.21,33.27 v61.21,33.91 | C30.2 34.54,22.42 U$2.31 34.54,26.29 33.27,27.56 29.46,27.56 28.19,26.29 28.19,22.48 28.83,21.84 28.83,14.59 | 66.93,6.43 66.93,15.21 I2C_EXPA.P$3 | 53.64,5.38 53.64,12.64 R8.1 arc90 52.01,12.95 C28.1 46.92,14.22 39.94,14.22 C27.1 39.62,13.59 | 0.89,17.68 0.89,7.87 C44.- 6.6,6.6 7.24,5.97 7.24,4.7 8.51,3.43 8.51,0.89 35.81,0.89 38.35,3.43 38.35,4.7 39.62,5.97 U$2.12 39.62,13.59 | ICSP.P$3 0.89,17.68 | MAIN_MCU_PWR.P$1 7.96,27.47 6.92,28.51 | 6.92,28.51 6.6,28.83 5.33,28.83 | 5.33,28.83 4.7,28.83 4.06,28.19 4.06,24.38 2.79,23.11 0.89,23.11 0.89,17.68 | Q13.2 Q17.2 21.84,19.67 C32.2 22.42,14.59 Q20.2 28.83,14.59 | 28.83,14.59 Q19.2 | 39.62,13.59 35.18,13.59 34.22,14.54 C29.2 C30.2 | Q12.2 35.99,22.1 C30.2 | v69.47,27.56 69.47,30.73 | D14.A v18.03,38.35 | C3.2 13.59,39.94 | C3.2 10.41,39.94 v10.41,38.35 | D10.A 12.95,37.08 C3.2 | SH1.1 5.33,28.83 | C5.2 6.92,28.51 | v43.43,35.81 42.8,35.81 42.8,43.43 47.45,43.43 | 47.45,43.43 v47.88,43.43 | BLUETOOTH.P$1 47.45,42.16 | 47.45,42.16 47.45,43.43
  Bottom 0.406: 66.93,4.7 66.29,5.33 60.21,5.33
  Bottom 0.61: 76.45,8.19 C39.2 | 76.45,17.4 v75.18,17.4 | v73.91,42.16 C7.2 | 43.12,35.81 v43.43,35.81
  pour Bottom (isolate 0.406): -0.38,-0.38 -1.02,30.73 6.6,30.73 7.24,43.43 24.38,43.43 24.38,33.91 33.27,30.73 37.08,27.56 42.16,27.56 42.16,47.24 78.99,46.61 78.36,-0.38
  pour Top (isolate 0.406): -1.02,30.73 6.6,30.73 6.6,38.99 11.68,38.99 12.32,43.43 24.38,43.43 24.38,34.54 32,31.37 37.08,27.56 42.16,27.56 42.16,47.24 78.99,46.61 78.36,-0.38 -1.65,-1.65
ICSP_MCLR
  Bottom 0.406: ICSP.P$1 7.78,13.68 U$2.1
  Bottom 0.61: U$2.1 R43.2
ICSP_PGC
  Bottom 0.406: U$2.39 11.68,22.48 6.6,22.48 6.4,22.27 ICSP.P$5
ICSP_PGD
  Bottom 0.406: U$2.40 10.41,23.75 6.22,23.75 4.95,22.48 4.95,20.57 5.84,19.68 ICSP.P$4
ICSP_VCC
  Bottom 0.406: U$2.32 32,22.42 C30.1 | C30.1 32.64,21.78 | ICSP.P$2 2.98,15.68 D6.C 2.16,14.86 1.52,14.22 1.52,9.78 7.87,9.78 7.87,6.6 8.51,5.97 8.51,4.7 9.78,3.43 9.78,1.52 35.18,1.52 37.08,3.43 U$2.11 37.08,11.89 36.45,12.52 33.91,12.52 32.32,14.11 C29.1 C30.1
KBRD_BUT1  (via drill 0.6)
  Top 0.406: v34.54,7.87 14.86,7.87 11.68,4.7
  Top 0.61: 11.68,4.7 v11.68,4.06
  Bottom 0.406: v34.54,7.87 U$2.10 | 16.13,5.33 13.59,5.33 12.32,4.06
  Bottom 0.61: 12.32,4.06 v11.68,4.06
  Bottom 0.813: KBRD.P$10 16.13,4.18 16.13,5.33
KBRD_BUT2
  Bottom 0.406: U$2.6 26.45,7.71
  Bottom 0.61: 26.45,7.71 KBRD.P$5
KBRD_BUT3
  Bottom 0.406: U$2.7 28.45,8.25
  Bottom 0.61: 28.45,8.25 KBRD.P$4
KBRD_BUT4
  Bottom 0.406: 30.45,8.79 U$2.8
  Bottom 0.61: KBRD.P$3 30.45,8.79
KBRD_BUT5
  Bottom 0.61: 32,4.3 U$2.9
  Bottom 0.813: KBRD.P$2 32,4.3
KBRD_EQU_BUT  (via drill 0.6)
  Top 0.406: v49.15,7.24 48.51,7.87 38.35,7.87 37.08,6.6 14.86,6.6 12.95,4.7 12.95,2.79
  Top 0.61: 12.95,2.79 v11.68,2.79
  Bottom 0.406: v49.15,7.24 47.24,9.14 U$2.15
  Bottom 0.61: KBRD.P$11 14.02,2.79 v11.68,2.79
KBRD_EQU_DOWN
  Bottom 0.406: U$2.4 22.45,6.63
  Bottom 0.61: 22.45,6.63 KBRD.P$7
KBRD_EQU_UP
  Bottom 0.406: U$2.5 24.45,7.17
  Bottom 0.61: 24.45,7.17 KBRD.P$6
KBRD_INT
  Bottom 0.406: 34.54,5.33 35.81,6.6 35.81,11.05 35.18,11.68 32.64,11.68 30.99,13.59 30.99,23.75 U$2.33
  Bottom 0.61: 34.54,3.95 34.54,5.33
  Bottom 0.813: KBRD.P$1 34.54,3.95
KBRD_VOL_DOWN
  Bottom 0.406: U$2.2 18.45,5.55
  Bottom 0.813: 18.45,5.55 KBRD.P$9
KBRD_VOL_UP
  Bottom 0.406: U$2.3 20.45,6.09
  Bottom 0.61: 20.45,6.09 KBRD.P$8
MKB_4.8V  (via drill 0.6)
  Top 0.406: R4.2 68.2,10.73 v68.2,12.32 | L1.2 62.48,39.56 R41.1 63.43,37.08 66.29,37.08 66.29,31.37 70.99,31.37 73.28,29.08 73.28,28.19 75.18,26.29 75.18,25.65 76.45,24.38 76.45,21.84 72.01,17.4 v68.2,17.4
  Top 0.61: v68.2,12.32 D7.A
  Bottom 0.406: v68.2,17.4 v68.2,12.32
MKB_PIC_PGD_PIN
  Bottom 0.406: R1.2 U$2.24
MKB_PIC_PGD_PIN_  (via drill 0.6)
  Top 0.406: v65.02,34.54 65.02,32 62.48,29.46 v60.58,29.46
  Bottom 0.406: R8.2 R1.1 53.59,20.26 53.59,26.29 52.96,26.92 52.32,26.92 52.32,27.56 53.59,28.83 55.5,28.83 56.13,29.46 v60.58,29.46 | v65.02,34.54 65.02,40.89 MKB_ICSP.4
MKB_PWR_ON_OFF
  Bottom 0.406: U$2.19 55.5,7.87 55.5,7.43 Q6.1
MKB_RX  (via drill 0.6)
  Top 0.406: MKB_UART.2 52.96,42.8 54.86,40.89 v56.13,40.89
  Bottom 0.61: v56.13,40.89 IC1.5
MKB_TX  (via drill 0.6)
  Top 0.406: v49.78,35.81 49.78,43.43
  Top 0.813: 49.78,43.43 MKB_UART.1
  Bottom 0.406: IC1.14 53.59,35.81 v49.78,35.81
N$1  (via drill 0.6)
  Top 0.406: R12.1 46.29,28.51 v45.34,27.56
  Bottom 0.406: R32.2 43.43,27.33 L4.1 43.16,27.56 v45.34,27.56
N$2
  Bottom 0.406: Q19.3 27.73,21.67 26.92,22.48 24.38,22.48 23.11,23.75 R3.P$5 23.22,28.93 D9.A
N$3
  Bottom 0.61: 33.27,41.4 29.97,41.4 28.19,39.62 R3.P$8
  Bottom 0.813: TO_MKB_ANT_POS_1450_1475.1 33.27,41.4 33.15,41.4
N$4
  Bottom 0.61: R3.P$7 28.19,33.91 30.46,33.91 37.08,29.46 | L3.2 37.08,27.83 37.08,29.46 | DAB_ANT.2 37.08,29.46
N$5
  Bottom 0.61: R3.P$9 32.64,34.54 38.35,34.54 FM_ANT.2
N$6
  Bottom 0.406: D5.A 23.11,34.01 R3.P$6 21.84,36.45 21.21,35.81 21.21,28.83 20.57,28.19 20.57,22.7 23.92,19.35 Q20.3
N$7
  Top 0.406: R2.1 62.48,6.6 61.21,5.33 59.43,5.33 Q2.3
N$8  (via drill 0.6)
  Top 0.406: R16.2 65.34,25.33 v63.75,23.75 | v56.13,26.67 56.13,21.84 55.5,21.21 v40.89,21.21
  Bottom 0.406: v63.75,23.75 63.12,23.75 63.12,25.65 61.21,27.56 57.4,27.56 v56.13,26.67 | v40.89,21.21 39.62,23.75 U$2.29
N$9  (via drill 0.6)
  Top 0.406: D3.C D7.C D11.C
  Top 0.61: v71.37,8.51
  Top 0.813: v71.37,8.51 D11.C
  Bottom 0.406: C39.1 72.96,10.09
  Bottom 0.813: Q3.3 v71.37,8.51 72.96,10.09
N$10  (via drill 0.6)
  Top 0.406: R14.2 71.37,28.19 70.1,29.46 65.02,29.46 63.75,28.19 v63.75,26.92 | v54.23,27.18 53.59,26.29 53.59,23.11 52.96,22.48 29.46,22.48 28.19,23.75 28.19,26.29 27.3,27.18 v26.29,27.18
  Bottom 0.406: v63.75,26.92 62.48,28.19 55.5,28.19 v54.23,27.18 | U$2.34 26.92,26.54 v26.29,27.18
N$12
  Bottom 0.406: L4.2 L3.1
N$13
  Bottom 0.406: R39.1 R7.1 61.53,20.26 62.48,21.21 64.77,21.21 66.04,22.48 66.04,28.83 65.28,29.59 63.75,29.59 61.85,31.62 59.94,31.62 IC1.9
N$15
  Bottom 0.406: Q7.2 42.16,6.48 U$2.13 arc-90 41.84,10.1 C27.2
N$16
  Bottom 0.406: Q7.1 44.7,5.21 U$2.14 44.7,12.63 arc-90 C28.2
N$17
  Bottom 0.406: U$2.20 59.94,12.57 R11.2
N$18
  Top 0.406: R4.1 63.75,9.14 61.21,6.6 58.67,6.6 57.4,5.33 55.62,5.33 Q15.3
N$19  (via drill 0.6)
  Top 0.406: 58.29,2.95 Q2.1
  Top 0.813: v58.29,2.16 58.29,2.95
  Bottom 0.406: 58.29,3.27 Q8.3
  Bottom 0.813: v58.29,2.16 58.29,3.27
N$20
  Bottom 0.406: Q12.3 39.62,20.52 39.62,19.3 38.35,18.67 35.81,18.67 35.81,15.49 36.18,15.13 Q16.1
N$21
  Top 0.406: R23.2 LED4.A
N$23
  Top 0.406: R12.2 43.43,30.73 LED6.A@1
N$25
  Bottom 0.406: Q17.3 18.03,20.62 18.03,26.29 17.4,26.92 16.76,26.92 16.76,29.83 Q18.1
N$26  (via drill 0.6)
  Top 0.406: R13.1 18.67,42.8 19.3,41.53 19.3,37.72 v18.03,36.45
  Bottom 0.406: R29.2 R22.1 16.13,36.45 v18.03,36.45
N$27
  Top 0.406: R13.2 12.95,42.8 LED7.A@1
N$28  (via drill 0.6)
  Top 0.813: Q14.1 v50.67,2.16
  Bottom 0.406: 50.67,3.27 Q5.3
  Bottom 0.813: v50.67,2.16 50.67,3.27
N$29
  Bottom 0.406: L5.1 arc-90 12.95,43.75 C3.1 15.49,41.84 D14.C 15.49,38.67 arc90 R22.2
N$30
  Bottom 0.406: L5.2 10.73,43.43 12V_DAB_FM_CONVERTER.1
N$31
  Top 0.406: R60.2 LED2.A
N$32
  Top 0.406: R25.1 64.39,11.68 60.58,7.87 57.4,7.87 56.13,6.6 53.08,6.6 Q14.3
N$33
  Bottom 0.406: Q16.3 39.82,16.45 R32.1
N$34
  Bottom 0.406: Q9.3 11.22,31.22 R28.1
N$35
  Bottom 0.406: Q18.3 15.66,31.22 R29.1
N$37  (via drill 0.6)
  Top 0.406: v54.48,2.16 54.5,2.17
  Top 0.813: 54.5,2.17 Q15.1
  Bottom 0.406: Q6.3 54.48,3.27
  Bottom 0.813: 54.48,3.27 v54.48,2.16
N$39
  Top 0.406: LED1.A 62.58,36.03 R41.2
N$41
  Bottom 0.406: R43.1 13.27,16.76 D8.C
N$42
  Bottom 0.61: D8.A 17.4,12.96 | 17.4,12.96 18.67,12.96 | 18.67,12.96 21.53,12.96 arc90 C32.1 | D4.A 18.77,13.06 arc90 18.67,12.96 | R44.2 17.08,13.27 arc-90 17.4,12.96
N$44
  Bottom 0.406: VM3.P$6 74.69,30.1 74.55,30.1 74.23,30.41 R20.1
N$47
  Bottom 0.406: R38.1 R6.1 58.67,20.26 58.67,26.29 59.31,26.92 60.58,26.92 61.85,25.65 61.85,22.48 65.02,22.48 65.02,27.56 63.75,28.83 63.12,28.83 61.21,30.73 59.31,30.73 58.67,31.37 IC1.10
N$85
  Bottom 0.406: Q13.3 13.12,21.38 15.49,23.75 15.49,26.29 14.86,26.92 12.32,26.92 12.32,29.83 Q9.1
N$87  (via drill 0.6)
  Top 0.406: 8.51,31.37 8.82,31.37 R100.1 R101.1 12.95,31.69 v12.95,35.18
  Bottom 0.406: v12.95,35.18 12.95,33.59 R28.2
N$88
  Top 0.406: R100.2 LED3.A@1
N$91  (via drill 0.6)
  Top 0.406: R101.2 11.05,34.22 v11.05,35.18
  Bottom 0.406: C5.1 9.14,36.45 | 9.14,36.45 L2.1 | v11.05,35.18 11.05,36.45 | 11.05,36.45 D10.C | 9.14,36.45 11.05,36.45
N$92
  Bottom 0.406: 12V_A_ANT.1 L2.2
PIC_RX_HV  (via drill 0.6)
  Top 0.406: Q1.3 56.13,32.81 v56.13,30.73
  Bottom 0.305: 51.05,21.21 48.51,21.21
  Bottom 0.406: U$2.26 R17.2 47.56,22.16 48.51,21.21 | v56.13,30.73 54.86,29.46 52.96,29.46 51.05,27.56 51.05,21.21
PIC_TX_HV  (via drill 0.6)
  Top 0.406: v52.32,30.73 Q11.3
  Bottom 0.406: R19.2 U$2.25 49.78,27.56 52.32,30.1 v52.32,30.73
PS_RELAY_SUSTAIN
  Bottom 0.406: PS_RELAY_SUSTAIN.1 U$2.36
PS_SWITCH_ON_OFF
  Bottom 0.406: U$2.35 PS_SWITCH_ON_OFF.1
RX_LV  (via drill 0.6)
  Top 0.406: v53.59,30.73 53.59,33.32 Q1.2 R15.2
  Bottom 0.406: IC1.13 54.86,31.37 54.23,30.73 v53.59,30.73
SCL
  Bottom 0.406: U$2.18 R67.1 57.4,12.62 59,14.22 62.48,14.22 I2C_EXPA.P$2
SDA
  Bottom 0.305: 61.34,16.76 56.13,16.76
  Bottom 0.406: U$2.23 R68.1 56.13,22.16 56.13,16.76 | 61.34,16.76 61.34,17.53 63.02,19.21 I2C_EXPA.P$1
SWITCH_2_DAB_ANT  (via drill 0.6)
  Top 0.406: v44.7,19.94 v30.1,19.94
  Bottom 0.406: U$2.27 v44.7,19.94 | v30.1,19.94 29.93,19.77 Q19.1
SWITCH_2_FM_ANT  (via drill 0.6)
  Top 0.406: v40.26,18.03 v26.29,18.03
  Bottom 0.406: U$2.28 42.16,19.94 v40.26,18.03 | v26.29,18.03 26.29,16.66 Q20.1
TO_MKB_VCC
  Top 0.61: L1.1 MKB_ICSP.2
TX_LV  (via drill 0.6)
  Top 0.406: Q11.2 R18.2 51.05,38.04 v51.05,40.89
  Bottom 0.406: IC1.3 53.59,40.26 52.96,40.89 v51.05,40.89
VDIAG
  Top 0.406: R29-FAKE.1 72.01,23.43 | 72.01,23.43 R14.1 | MCU_AMP.1 72.01,23.43
VM3_4.8V  (via drill 0.6)
  Top 0.406: R25.2 66.61,13.27 68.83,15.49 69.47,15.49 D3.A 69.47,15.49 | 74.55,33.91 74.55,28.19 v76.45,26.29 | R60.1 72.01,34.86
  Top 0.61: 69.47,15.49 v70.74,15.49 | 74.55,33.91 v72.01,33.91 72.01,34.86
  Bottom 0.406: 71.37,15.49 76.45,20.57 v76.45,26.29 | 74.4,33.91 VM3.P$3 | C7.1 73.91,33.91 73.28,33.91
  Bottom 0.61: v70.74,15.49 71.37,15.49 | v72.01,33.91 73.28,33.91 74.4,33.91
VM3_PWR_ON_OFF
  Bottom 0.406: U$2.17 52.32,8.07 Q5.1
VM3_RX
  Bottom 0.406: IC1.4 54.86,36.45 61.85,36.45 64.77,32.89 75.39,32.89 VM3.P$4
VM3_TX
  Bottom 0.406: IC1.11 57.4,35.18 61.85,35.18 64.23,32.16 74.39,32.16 VM3.P$5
